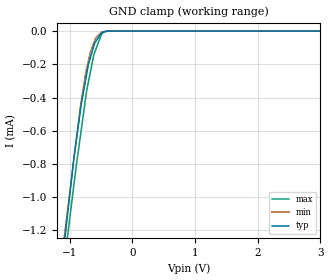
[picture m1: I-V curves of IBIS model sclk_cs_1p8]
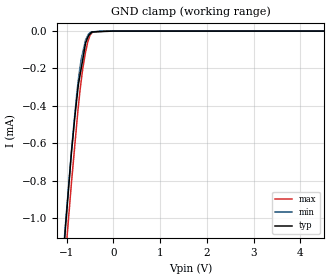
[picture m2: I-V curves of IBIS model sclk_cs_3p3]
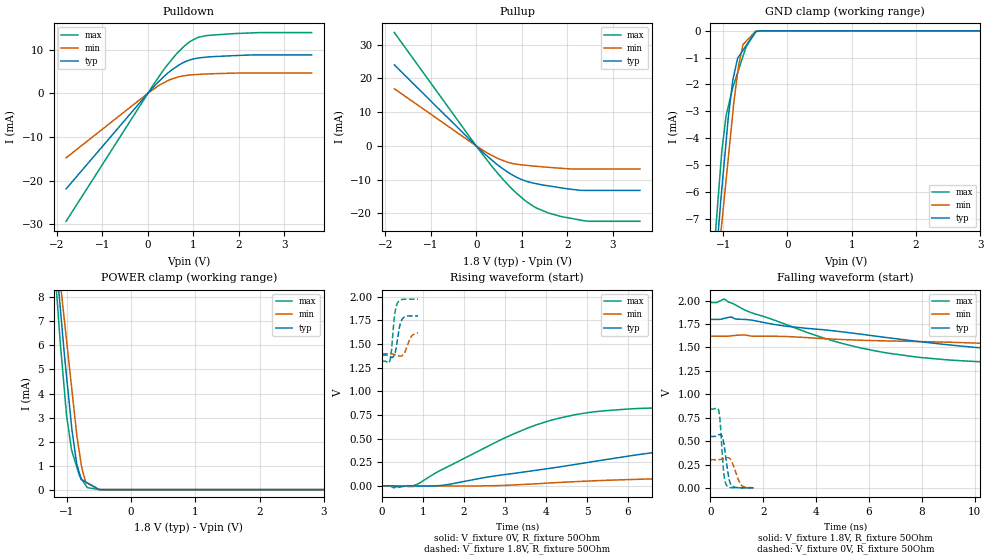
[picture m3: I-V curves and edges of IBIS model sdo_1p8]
|Texas Instruments Incorporated
| 1.2V, 10 bit 240KSPS, Serial ADC
| Marketing part#   Digital Voltage Range   Package-type   #pins
| ADS7867IDBVR   1.2V - 3.6V   SOT-23   6
| ADS7867IDBVRG4   1.2V - 3.6V   SOT-23   6
| ADS7867IDBVT   1.2V - 3.6V   SOT-23   6
| ADS7867IDBVTG4   1.2V - 3.6V   SOT-23   6
[IBIS Ver]   3.2
[File name]   ads7867.ibs
|SIMDE Ver   V3.0 - 201101 - RHL4 - Build 457
[File Rev]   1.0
[Date]   6/15/2011
[Source]
| Texas Instruments Incorporated.
| Analog-eLab Design Center, HPA
| 12500 TI Blvd
| Dallas, TX -75243
| e-mail: elab_ibis@list.ti.com
[Notes]   Revision History:
| Rev 1.0: 6/15/2011
| - Initial version of the model
| - Model generated from simulations in TISPICE
| - Model matched to SPICE simulation
| - C_comp although listed in numerical order of value are
|   obtained from varying PVT conditions. For PVT conditions for
|   each specific value refer the buffer description under
|   respective [Model]. IBIS model user is responsible for using
|   appropriate C_comp to simulate for Signal Integrity.
| - Model names with a trailing _1p8 contains the model for
|   1.8V [1.62V and 1.98V].Model names with a trailing _3p3
|   contains the model for 3.3V [3.0V and 3.6V].
| - Relative part of ADS7866.
[Disclaimer]
| This model is designed as an aid for customers of Texas Instruments.
| TI and its licensors and suppliers make no warranties, either expressed
| or implied, with respect to this  model, including the warranties of
| merchantability or fitness for a particular purpose. The model is
| provided solely on an "as is" basis. The entire risk as to its quality
| and performance is with the customer.
[Copyright]
 (C) Copyright 2011 Texas Instruments Incorporated.All rights reserved.
|   ADS7867
[Component]   ADS7867
[Manufacturer]   TI
[Package]   |6 SOT-23   -  DBV package
|   typ   min   max
R_pkg   0.05459   0.04615   0.06295
L_pkg   1.54446nH   1.37485nH   1.73255nH
C_pkg   0.23361pF   0.14419pF   0.28060pF
[Pin]  signal_name   model_name   R_pin   L_pin   C_pin
1   REF/VDD   POWER   0.05091   1.87896nH  0.29369pF
2   GND   GND   0.05056   1.89176nH  0.29842pF
3   VIN   TERM   0.05449   1.73255nH  0.28060pF
4   SCLK   SCLK_CS   0.04615   1.37485nH  0.24252pF
5   SDO   SDO   0.05476   1.68868nH  0.26714pF
6   _CS   SCLK_CS   0.06295   1.38176nH  0.14419pF
|   Model Selectors
[Model Selector] SCLK_CS
sclk_cs_1p8  1.8V digital input
sclk_cs_3p3  3.3V digital input
[Model Selector] SDO
sdo_1p8  1.8V digital 3-state output
sdo_3p3  3.3V digital 3-state output
[Model Selector] TERM
term_1-8V  1.8V nominal termination
term_3-3V  3.3V nominal termination
[Model] term_1-8V
Model_type Terminator
C_comp   1.0e-20F  1.0e-20F  1.0e-20F
|   typ   min   max
[Voltage Range]   1.8V   1.62V   1.98V
[POWER Clamp Reference]   1.8V   1.62V   1.98V
[GND Clamp Reference]   0V   0V   0V
|Ambient Temperature   25   85   -40
|Junction Temperature
[Temperature Range]   27   87   -40
[Model] term_3-3V
Model_type Terminator
C_comp   1.0e-20F  1.0e-20F  1.0e-20F
|   typ   min   max
[Voltage Range]   3.3V   3.0V   3.6V
[POWER Clamp Reference]   3.3V   3.0V   3.6V
[GND Clamp Reference]   0V   0V   0V
|Ambient Temperature   25   85   -40
|Junction Temperature
[Temperature Range]   27   87   -40
| Models and submodels in the file (6): sclk_cs_1p8 (Input), sclk_cs_3p3 (Input), sdo_1p8 (3-state), sdo_3p3 (3-state), term_1-8V (Terminator), term_3-3V (Terminator)
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|   sclk_cs_1p8 Model
[Model]   sclk_cs_1p8
Model_type   Input
Vinl = 0.54
Vinh = 1.26
|   typ   min   max
|   (nom PVT)   (fast PVT)   (slow PVT)
|C_comp from frequency sweep method (F=3.4MHz)
|Average
|C_comp   7.572e-13   7.532e-13   7.634e-13
|C_comp from LC tank measurement(L=1nH)
|Average
|Resonant Frequency(Hz)   8.010e+09   8.110e+09   7.900e+09
C_comp   3.952e-13   3.855e-13   4.063e-13
| Where nom  PVT is Nominal Process, 1.8V, 27C
|   Fast PVT is Strong Process,  1.98V, -40C
|   Slow PVT is Weak Process,   1.62V, 87C
[Model Spec]
Vinl   0.54   0.324   0.594
Vinh   1.26   1.134   1.386
[Voltage Range]   1.8   1.62   1.98
|Ambient Temperature   25   85   -40
|Junction Temperature
[Temperature Range]   27   87   -40
[Power Clamp Reference]   1.8   1.62   1.98
[GND Clamp Reference]   0   0   0
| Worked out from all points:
|   GND clamp passes 1 mA (typ) near -1.00 V on its own axis
[GND Clamp]
|   Voltage   I(typ)   I(min)   I(max)
-1.8V     -3.949mA   -3.627mA   -4.226mA
-1.097V   -1.315mA   -1.269mA   -1.425mA
-932.4mV  -759.3uA   -767.3uA   -920.7uA
-832.7mV  -487.8uA   -462.9uA   -639.8uA
-813.6mV  -436.1uA   -416.5uA   -587.5uA
-730.6mV  -261.9uA   -225.5uA   -360.2uA
-700.2mV  -198.8uA   -176.2uA   -301.8uA
-665.8mV  -154.5uA   -120.9uA   -237uA
-603mV    -73.59uA   -58.74uA   -129.7uA
-494.1mV  -11.16uA   -7.499uA   -20.1uA
-350.5mV  -275.4nA   -331.7nA   -169.1nA
3.6V      0A         0A         0A
[POWER Clamp]
|   Voltage   I(typ)   I(min)   I(max)
-1.8V     0A         0A         0A
3.6V      0A         0A         0A
|   sclk_cs_3p3 Model
[Model]   sclk_cs_3p3
Model_type   Input
Vinl = 0.8
Vinh = 2
|   typ   min   max
|   (nom PVT)   (fast PVT)   (slow PVT)
|C_comp from frequency sweep method (F=3.4MHz)
|Average
|C_comp   7.283e-13   7.258e-13   7.358e-13
|C_comp from LC tank measurement(L=1nH)
|Average
|Resonant Frequency(Hz)   8.000e+09   8.090e+09   7.900e+09
C_comp   3.962e-13   3.874e-13   4.063e-13
| Where nom  PVT is Nominal Process, 3.3V, 27C
|   Fast PVT is Strong Process,  3.6V, -40C
|   Slow PVT is Weak Process,   3V, 87C
[Voltage Range]   3.3   3   3.6
|Ambient Temperature   25   85   -40
|Junction Temperature
[Temperature Range]   27   87   -40
[Power Clamp Reference]   3.3   3   3.6
[GND Clamp Reference]   0   0   0
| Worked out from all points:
|   GND clamp passes 1 mA (typ) near -1.01 V on its own axis
[GND Clamp]
|   Voltage   I(typ)   I(min)   I(max)
-3.3V     -9.423mA   -8.546mA   -10.44mA
-1.038V   -1.103mA   -1.079mA   -1.25mA
-1.02V    -1.039mA   -1.023mA   -1.194mA
-897.6mV  -657.2uA   -646.1uA   -818uA
-821.7mV  -455.8uA   -441.5uA   -606.2uA
-735mV    -268.9uA   -233.9uA   -372.6uA
-662.4mV  -164.2uA   -123.6uA   -217.3uA
-601.2mV  -75.93uA   -55.6uA    -122.2uA
-543.6mV  -32.5uA    -22.6uA    -55.38uA
-480mV    -10.25uA   -5.513uA   -16.22uA
-133.2mV  -1.35uA    -18.61nA   0A
6.6V      0A         0A         0A
[POWER Clamp]
|   Voltage   I(typ)   I(min)   I(max)
-3.3V     0A         0A         0A
6.6V      0A         0A         0A
|   sdo_1p8 Model
[Model]   sdo_1p8
Model_type   3-state
Polarity   Non-Inverting
Vmeas = 0.9
Vref = 0.9
Cref = 2pF
Rref = 50
|   typ   min   max
|   (nom PVT)   (fast PVT)   (slow PVT)
|C_comp from frequency sweep method (F=1.7MHz)
|C_comp   4.540e-12   2.844e-12   5.993e-12
|ON state : BUFFER OUTPUT TURNED HIGH
|C_comp   4.540e-12   2.844e-12   5.993e-12
|OFF state: BUFFER IN HIGH IMPEDANCE
|C_comp   7.638e-13   7.544e-13   7.728e-13
|C_comp from LC tank measurement(L=1nH)
|Resonant Frequency(Hz)   6.420e+09   6.430e+09   6.380e+09
C_comp   6.152e-13   6.133e-13   6.229e-13
|ON state : BUFFER OUTPUT TURNED HIGH
|Resonant Frequency(Hz)   6.420e+09   6.430e+09   6.380e+09
|C_comp   6.152e-13   6.133e-13   6.229e-13
|OFF state: BUFFER IN HIGH IMPEDANCE
|Resonant Frequency(Hz)   6.580e+09   6.610e+09   6.550e+09
|C_comp   5.856e-13   5.803e-13   5.910e-13
| Where nom  PVT is Nominal Process, 1.8V, 27C
|   Fast PVT is Strong Process,  1.98V, -40C
|   Slow PVT is Weak Process,   1.62V, 87C
[Voltage Range]   1.8   1.62   1.98
|Ambient Temperature   25   85   -40
|Junction Temperature
[Temperature Range]   27   87   -40
[Pullup Reference]   1.8   1.62   1.98
[Pulldown Reference]   0   0   0
[Power Clamp Reference]   1.8   1.62   1.98
[GND Clamp Reference]   0   0   0
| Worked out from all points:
|   slope of the pulldown table from 0 to 0.27 V, typ, clamps not added: 90.2 ohm
|   slope of the pullup table from 0 to 0.27 V, typ, clamps not added: 80.8 ohm
|   GND clamp passes 1 mA (typ) near -0.77 V on its own axis
|   POWER clamp passes 1 mA (typ) near -0.84 V on its own axis
|   falling waveform, V_fixture 1.8V, R_fixture 50Ohm: 20-80 % time 8.42ns typ, 15.2ns min, 4.68ns max; typ from 1.8 V to 1.38 V
|   rising waveform, V_fixture 0V, R_fixture 50Ohm: 20-80 % time 5.53ns typ, 10.9ns min, 2.52ns max; typ from 0 V to 0.55 V
|   rising waveform, V_fixture 1.8V, R_fixture 50Ohm: 20-80 % time 99.7ps typ, 123ps min, 85.8ps max; typ from 1.38 V to 1.8 V
|   falling waveform, V_fixture 0V, R_fixture 50Ohm: 20-80 % time 168ps typ, 237ps min, 126ps max; typ from 0.55 V to 0.001 V
[Pulldown]
|   Voltage   I(typ)   I(min)   I(max)
-1.8V     -21.89mA   -14.78mA   -29.31mA
20.08fV   5.501pA    6.118pA    6.615pA
180mV     2.084mA    1.33mA     2.865mA
378.2mV   4.086mA    2.553mA    5.838mA
601.9mV   5.892mA    3.516mA    8.695mA
855.4mV   7.379mA    4.097mA    11.27mA
1.093V    8.024mA    4.293mA    12.74mA
1.307V    8.28mA     4.411mA    13.22mA
2.479V    8.777mA    4.645mA    13.88mA
3.6V      8.777mA    4.645mA    13.88mA
[GND Clamp]
|   Voltage   I(typ)   I(min)   I(max)
-1.8V     -30.58mA   -28.47mA   -33.91mA
-1.108V   -8.464mA   -9.41mA    -7.171mA
-1.037V   -6.318mA   -7.54mA    -4.973mA
-1.022V   -5.917mA   -7.177mA   -4.507mA
-952.4mV  -4.078mA   -5.51mA    -3.138mA
-918mV    -3.178mA   -4.684mA   -2.794mA
-851.4mV  -1.867mA   -3.082mA   -2.127mA
-758.2mV  -961.6uA   -1.274mA   -1.438mA
-691.7mV  -725.1uA   -513uA     -949.6uA
-643.5mV  -553.3uA   -391.4uA   -594.7uA
-494.1mV  -24.03uA   -14.83uA   -45.72uA
3.6V      0A         0A         0A
[Pullup]
|   Voltage   I(typ)   I(min)   I(max)
-1.8V     24.03mA    16.95mA    33.6mA
20.08fV   -11.19pA   -15.79pA   -10.94pA
218.7mV   -2.748mA   -1.887mA   -3.869mA
432.5mV   -5.222mA   -3.441mA   -7.471mA
686.9mV   -7.723mA   -4.813mA   -11.34mA
894.6mV   -9.342mA   -5.446mA   -14.11mA
1.063V    -10.29mA   -5.702mA   -16.09mA
1.315V    -11.19mA   -6.036mA   -18.34mA
1.59V     -11.85mA   -6.351mA   -19.91mA
1.869V    -12.44mA   -6.635mA   -20.94mA
2.376V    -13.19mA   -6.866mA   -22.2mA
3.6V      -13.19mA   -6.866mA   -22.35mA
[POWER Clamp]
|   Voltage   I(typ)   I(min)   I(max)
-1.8V     30.26mA    28.19mA    33.57mA
-1.201V   10.64mA    11.41mA    9.821mA
-1.111V   7.918mA    8.914mA    6.541mA
-1.099V   7.54mA     8.606mA    6.085mA
-1.033V   5.54mA     6.979mA    4.054mA
-999.9mV  4.654mA    6.155mA    3.046mA
-924.7mV  2.652mA    4.292mA    1.654mA
-846mV    1.112mA    2.344mA    964.4uA
-769.5mV  414.9uA    961.9uA    436.8uA
-679.1mV  278.7uA    272.6uA    82.31uA
-495mV    1.102uA    3.511uA    317.3nA
3.6V      0A         0A         0A
[Ramp]
R_load = 50
|   typ   min   max
dV/dt_r   0.330165/5.52951e-09   0.181383/1.08672e-08   0.5053/2.52165e-09
dV/dt_f   0.250234/8.40099e-09   0.133146/1.50658e-08   0.39693/4.6875e-09
[Falling Waveform]
V_fixture = 1.8V
V_fixture_min = 1.62V
V_fixture_max = 1.98V
R_fixture = 50Ohm
|   Time   V(typ)   V(min)   V(max)
0s        1.8V       1.62V      1.98V
537ps     1.812V     1.619V     2.015V
1.616ns   1.79V      1.621V     1.865V
4.213ns   1.691V     1.596V     1.608V
5.708ns   1.641V     1.577V     1.494V
7.739ns   1.568V     1.564V     1.4V
10.09ns   1.499V     1.546V     1.349V
13.95ns   1.431V     1.503V     1.324V
20.12ns   1.393V     1.448V     1.319V
50ns      1.383V     1.398V     1.318V
[Rising Waveform]
V_fixture = 0V
V_fixture_min = 0V
V_fixture_max = 0V
R_fixture = 50Ohm
|   Time   V(typ)   V(min)   V(max)
0s        404.7pV    655.5pV    357.2pV
820ps     -1.025mV   -2.92mV    10.2mV
2.979ns   118.9mV    5.09mV     504.7mV
4.014ns   180.6mV    28.68mV    680.4mV
5.047ns   249.7mV    51.47mV    776.5mV
6.169ns   325.3mV    68.49mV    817.1mV
8.892ns   460mV      109mV      839.6mV
13.1ns    533.5mV    191.6mV    842.2mV
20.11ns   549.3mV    273.8mV    842.2mV
35.84ns   550.3mV    301.5mV    842.2mV
[Rising Waveform]
V_fixture = 1.8V
V_fixture_min = 1.62V
V_fixture_max = 1.98V
R_fixture = 50Ohm
|   Time   V(typ)   V(min)   V(max)
0s        1.383V     1.398V     1.318V
150ps     1.379V     1.399V     1.299V
204ps     1.366V     1.398V     1.342V
229ps     1.362V     1.397V     1.429V
302ps     1.388V     1.39V      1.792V
377ps     1.554V     1.379V     1.935V
444ps     1.712V     1.373V     1.966V
517ps     1.777V     1.388V     1.974V
704ps     1.799V     1.573V     1.976V
878ps     1.798V     1.618V     1.974V
[Falling Waveform]
V_fixture = 0V
V_fixture_min = 0V
V_fixture_max = 0V
R_fixture = 50Ohm
|   Time   V(typ)   V(min)   V(max)
0s        550.3mV    302.3mV    842.2mV
324ps     567.3mV    302.2mV    822mV
373ps     571mV      304mV      706.3mV
459ps     542.4mV    309.3mV    332.8mV
512ps     475.7mV    313.8mV    155.5mV
616ps     264.8mV    322.5mV    27.28mV
715ps     89.72mV    318.4mV    6.515mV
816ps     21.7mV     279.7mV    3.144mV
1.171ns   1.844mV    31.32mV    1.636mV
1.635ns   926.9uV    1.878mV    917.2uV
